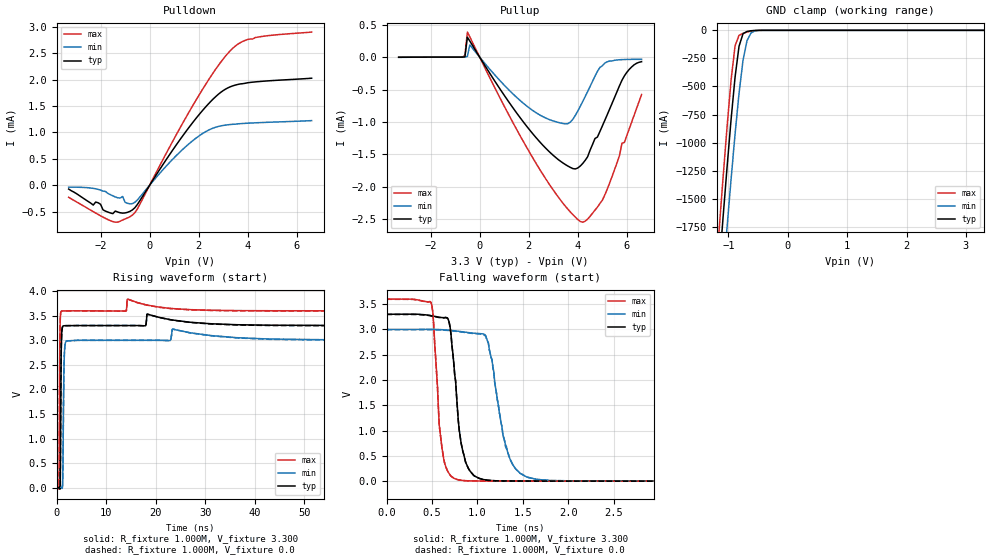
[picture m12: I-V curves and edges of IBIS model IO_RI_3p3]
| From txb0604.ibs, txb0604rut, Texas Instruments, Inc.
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|   Model IO_RI_3p3
[Model] IO_RI_3p3
Model_type 3-state
Polarity   Non-Inverting
Enable   Active-High
Vmeas =  1.650V
Cref =  0.100nF
Rref =  1.000M
Vref =  0.0V
C_comp   3.560pF   3.290pF   3.850pF
[Temperature Range]   27.000   0.125k   -40.000
[Voltage Range]   3.300V   3.000V   3.600V
[Pullup Reference]   3.300V   3.000V   3.600V
[Pulldown Reference]   0.0V   0.0V   0.0V
[POWER Clamp Reference]   3.300V   3.000V   3.600V
[GND Clamp Reference]   0.0V   0.0V   0.0V
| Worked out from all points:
|   slope of the pulldown table from 0 to 0.495 V, typ, clamps not added: 1.38 kohm
|   slope of the pullup table from 0 to 0.495 V, typ, clamps not added: 1.66 kohm
|   GND clamp passes 1 mA (typ) near -0.54 V on its own axis
|   rising waveform, R_fixture 1.000M, V_fixture 3.300: 20-80 % time 134ps typ, 189ps min, 103ps max; typ from 0.004 V to 3.3 V
|   rising waveform, R_fixture 1.000M, V_fixture 0.0: 20-80 % time 134ps typ, 189ps min, 103ps max; typ from 0 V to 3.29 V
|   falling waveform, R_fixture 1.000M, V_fixture 3.300: 20-80 % time 109ps typ, 168ps min, 80.5ps max; typ from 3.3 V to 0.004 V
|   falling waveform, R_fixture 1.000M, V_fixture 0.0: 20-80 % time 109ps typ, 168ps min, 80.6ps max; typ from 3.29 V to 0 V
[Pulldown]
-3.3V     -72.84uA   -36.07uA   -229.5uA
-2.3V     -376.5uA   -59.65uA   -501.2uA
-2.2V     -320.3uA   -67.87uA   -528.2uA
-1.5V     -539.4uA   -201.9uA   -690.2uA
-1.1V     -529.4uA   -214.4uA   -659.3uA
-800mV    -495.4uA   -353.9uA   -597.1uA
-500mV    -365.5uA   -279.3uA   -450uA
1.8V      1.215mA    860.7uA    1.544mA
2.7V      1.684mA    1.101mA    2.206mA
3.3V      1.87mA     1.152mA    2.558mA
4.3V      1.959mA    1.183mA    2.799mA
6.6V      2.029mA    1.225mA    2.904mA
[Pullup]
|Voltage   I(typ)   I(min)   I(max)
-3.3V     -2.098uA   -4.195uA   -1.345uA
-700mV    102.1nA    88.29nA    554.3nA
-600mV    5.216uA    242.9nA    27.24uA
-500mV    306.5uA    10.3uA     386.2uA
-400mV    247.3uA    188.8uA    311.9uA
1.4V      -804.7uA   -582.6uA   -1.04mA
2.8V      -1.445mA   -956.8uA   -1.938mA
3.6V      -1.681mA   -1.025mA   -2.347mA
4.2V      -1.64mA    -684.8uA   -2.546mA
5.1V      -975.2uA   -91.58uA   -2.126mA
5.9V      -288.4uA   -36.71uA   -1.315mA
6.6V      -69.89uA   -34.29uA   -576.7uA
[GND_clamp]
|Voltage   I(typ)   I(min)   I(max)
-3.3V     -15.16A    -14.83A    -15.52A
-1.156V   -2.118A    -2.633A    -1.775A
-1.089V   -1.661A    -2.187A    -1.307A
-1.022V   -1.216A    -1.75A     -856.6mA
-955mV    -794.8mA   -1.327A    -443.9mA
-888mV    -417.7mA   -925.5mA   -138.1mA
-821mV    -142.1mA   -561.7mA   -44.71mA
-754mV    -30.52mA   -267.7mA   -26.73mA
-687mV    -10.01mA   -92.37mA   -15.03mA
-620mV    -3.936mA   -24.04mA   -6.702mA
-553mV    -1.125mA   -4.87mA    -1.879mA
3.3V      0A         0A         0A
[Ramp]
| variable   typ   min   max
dV/dt_r   1.977/0.136n   1.796/0.190n   2.157/0.102n
dV/dt_f   1.977/0.108n   1.797/0.171n   2.158/77.002p
R_load = 1.000M
[Rising Waveform]
R_fixture= 1.000M
V_fixture= 3.300
V_fixture_min= 3.000
V_fixture_max= 3.600
|time   V(typ)   V(min)   V(max)
0s        4.455mV    5.332mV    3.941mV
510ps     8.11mV     4.54mV     21.52mV
640ps     -4.223mV   3.757mV    2.576V
730ps     30.58mV    4.869mV    3.344V
920ps     2.536V     9.881mV    3.584V
1.02ns    3.072V     2.442mV    3.593V
1.26ns    3.283V     227.5mV    3.596V
1.57ns    3.296V     2.689V     3.597V
1.97ns    3.298V     2.985V     3.598V
120ns     3.3V       3V         3.6V
[Rising Waveform]
R_fixture= 1.000M
V_fixture= 0.0
V_fixture_min= 0.0
V_fixture_max= 0.0
|time   V(typ)   V(min)   V(max)
0s        -4.254uV   10.8uV     -5.2uV
510ps     3.557mV    -783.1uV   16.25mV
640ps     -8.833mV   -1.6mV     2.573V
730ps     25.91mV    -546.1uV   3.343V
920ps     2.534V     4.345mV    3.584V
1.02ns    3.071V     -3.066mV   3.593V
1.26ns    3.283V     221.4mV    3.596V
1.58ns    3.296V     2.712V     3.597V
2ns       3.298V     2.987V     3.598V
120ns     3.295V     2.994V     3.595V
[Falling Waveform]
R_fixture= 1.000M
V_fixture= 3.300
V_fixture_min= 3.000
V_fixture_max= 3.600
|time   V(typ)   V(min)   V(max)
0s        3.3V       3V         3.6V
490ps     3.271V     3.001V     3.535V
580ps     3.241V     2.997V     1.109V
670ps     3.228V     2.987V     208.2mV
820ps     759.1mV    2.957V     19.38mV
960ps     114.2mV    2.925V     5.741mV
1.12ns    18.9mV     2.74V      3.887mV
1.42ns    3.993mV    246.1mV    2.595mV
2.2ns     1.846mV    3.469mV    1.161mV
120ns     4.466mV    5.34mV     3.951mV
[Falling Waveform]
R_fixture= 1.000M
V_fixture= 0.0
V_fixture_min= 0.0
V_fixture_max= 0.0
|time   V(typ)   V(min)   V(max)
0s        3.295V     2.994V     3.595V
490ps     3.265V     2.994V     3.531V
580ps     3.235V     2.991V     1.106V
670ps     3.222V     2.98V      207.8mV
820ps     757.2mV    2.95V      19.29mV
960ps     113.9mV    2.918V     5.685mV
1.12ns    18.8mV     2.734V     3.835mV
1.42ns    3.93mV     245.2mV    2.546mV
2.2ns     1.788mV    3.385mV    1.113mV
120ns     6.685uV    18.55uV    4.528uV
